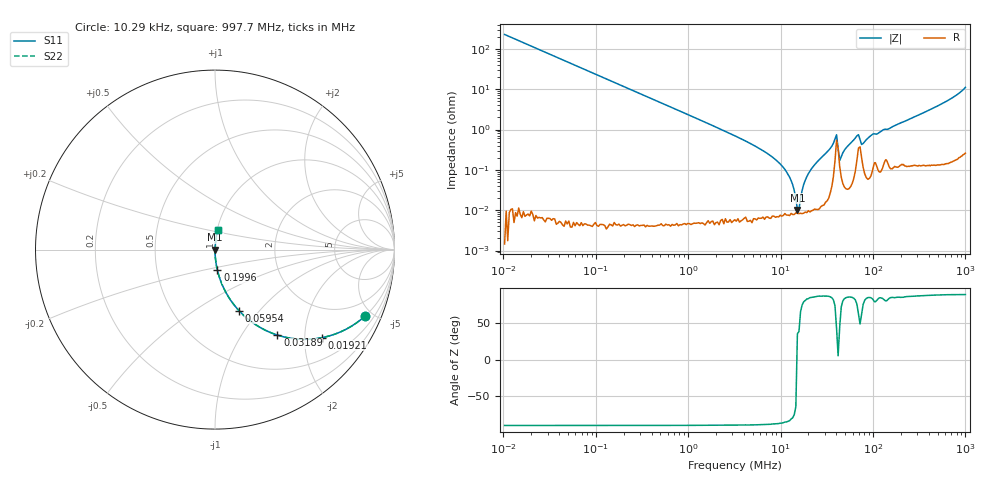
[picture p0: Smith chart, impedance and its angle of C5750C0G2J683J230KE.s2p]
! S-Parameter Data Generated by TDK Corporation
! Copyright(C) 2025 TDK Corporation.
! All Rights Reserved.
! TDK P/N: C5750C0G2J683J230KE (Multilayer Ceramic Chip Capacitor)
! Property: C=68nF
! Size(LxWxT): 5.7x5x2.3mm
! Model Type: s2p (Touchstone File Format Version 1.0)
! Frequency: DC=Yes Start=0.01028704MHz Stop=997.7393MHz 352points Log-sweep
! Model Generated on July 30, 2025
! Terms and conditions regarding TDK Simulation Models:
! 1)This simulation model is being provided solely for informational
!  purposes. Please refer to the specifications of the products in
!  terms of detailed characteristics of such products.
! 2)In no event shall TDK Corporation of any of its subsidiaries be
!  liable for any loss or damage arising, directly or indirectly,
!  from any information contained in this simulation model, including,
!  but not limited to loss or damages arising from any inaccuracies,
!  omissions or errors in connection with such information.
! 3)Any and all copyrights on this simulation model are owned by
!  TDK Corporation.  Duplication or redistribution of this simulation
!  model without prior written permission from TDK Corporation
!  is prohibited.
! 4)This simulation model is subject to any modification or change
!  without any prior notice.
! 5)Neither TDK Corporation nor any of its subsidiaries shall make any
!  warranty, express or implied, including but not limited to the
!  correctness, implied warranties of merchantability and fitness for
!  a particular purpose with respect to this simulation models.
! 6)The use of this simulation model shall be deemed to have consented
!  to the terms and conditions hereof.
! Port Assignments:
!  1 ---| |--- 2
! Applicable Conditions:
!  Temperature = 25 degC
!  DC Bias Voltage = 0 V
!  Small Signal Operation
# Hz S MA R 50
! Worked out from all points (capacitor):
!   351 points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, 10.29 kHz to 997.7 MHz, reference 50 ohm
!   read as one part in series: C = 68.3 nF near 10.7 kHz
!   lowest |Z| = 10.2 mohm at 15.17 MHz (marker M1)
!   series resonance near 15.03 MHz, so ESL is about 1.6 nH
!   S11 on the Smith chart (normalised r, x): 10.29 kHz: 1.00, -4.53; 19.21 kHz: 1.00, -2.43; 31.89 kHz: 1.00, -1.46; 59.54 kHz: 1.00, -0.78; 199.6 kHz: 1.00, -0.23; 997.7 MHz: 1.01, +0.22
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10287.04  0.9148 -23.8  0.4038 66.2  0.4038 66.2  0.9148 -23.8
19205.1  0.7717 -39.5  0.636 50.5  0.636 50.5  0.7717 -39.5
31893.81  0.5899 -53.8  0.8074 36.2  0.8074 36.2  0.5899 -53.8
59543.25  0.3644 -68.6  0.9312 21.4  0.9312 21.4  0.3644 -68.6
72370.14  0.3065 -72.1  0.9518 17.8  0.9518 17.8  0.3065 -72.1
199590.2  0.1159 -83.3  0.9932 6.7  0.9932 6.7  0.1159 -83.3
489646.8  0.04749 -87.2  0.9988 2.7  0.9988 2.7  0.04749 -87.2
3312886  0.006707 -89.2  0.9999 0.4  0.9999 0.4  0.006707 -89.2
1.067992e7  0.001152 -86.2  0.9999 0.1  0.9999 0.1  0.001152 -86.2
1.349709e7  0.0004263 -79.4  0.9999 0.0  0.9999 0.0  0.0004263 -79.4
1.517317e7  0.0001017 35.1  0.9999 -0.0  0.9999 -0.0  0.0001017 35.1
1.57769e7  0.0001052 38.3  0.9999 -0.0  0.9999 -0.0  0.0001052 38.3
1.773608e7  0.0004337 78.8  0.9999 -0.0  0.9999 -0.0  0.0004337 78.8
2.241455e7  0.001196 85.1  0.9999 -0.1  0.9999 -0.1  0.001196 85.1
3.442938e7  0.003416 85.3  0.9997 -0.2  0.9997 -0.2  0.003416 85.3
4.024488e7  0.007363 42.4  0.9946 -0.3  0.9946 -0.3  0.007363 42.4
4.351124e7  0.001697 44.0  0.9988 -0.1  0.9988 -0.1  0.001697 44.0
4.891449e7  0.003075 82.8  0.9996 -0.2  0.9996 -0.2  0.003075 82.8
6.949378e7  0.007415 61.7  0.9965 -0.4  0.9965 -0.4  0.007415 61.7
7.513403e7  0.004241 61.6  0.998 -0.2  0.998 -0.2  0.004241 61.6
1.49005e8  0.01048 82.8  0.9987 -0.6  0.9987 -0.6  0.01048 82.8
9.977393e8  0.1097 82.4  0.9914 -6.3  0.9914 -6.3  0.1097 82.4
